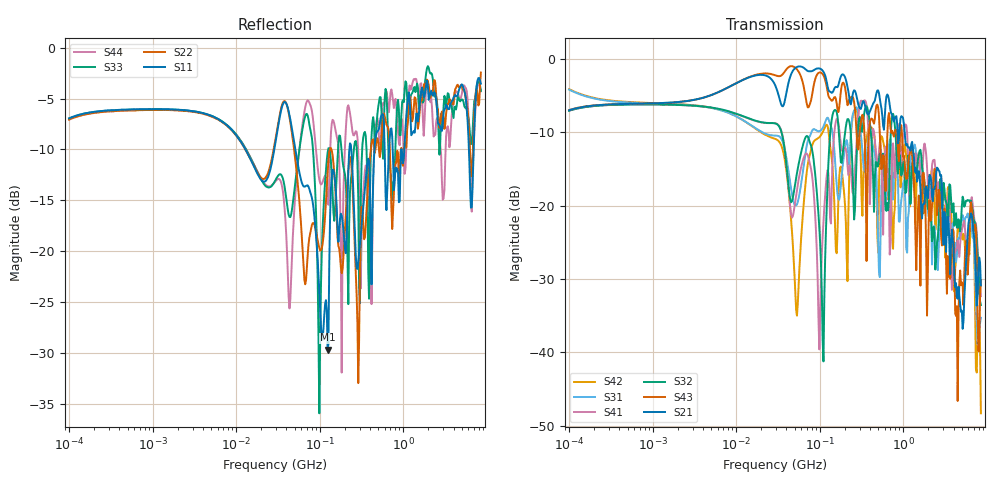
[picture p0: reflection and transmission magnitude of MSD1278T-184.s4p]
# MHz S MA R 50
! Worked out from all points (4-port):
!   498 points, 100 kHz to 8.5 GHz, reference 50 ohm
!   strongest paths, dB at 100 kHz, 1.698 MHz, 29.49 MHz, 500.7 MHz, 8.5 GHz:
!     S21: -7.0, -6.0, -3.7, -4.3, -30.9
!     S43: -7.0, -6.0, -2.3, -6.7, -30.2
!     S32: -7.1, -6.3, -8.8, -14.6, -33.5
!     S41: -7.1, -6.3, -8.8, -14.0, -32.3
!     S31: -4.2, -6.2, -10.5, -24.9, -35.3
!     S42: -4.2, -6.2, -10.9, -26.3, -48.3
!   lowest |S11| = -29.7 dB at 124.3 MHz (marker M1), VSWR 1.07, Z = 53.3 - j0.646 ohm
!   |S11| at or under -10 dB: 51.1 MHz to 226.3 MHz (175.2 MHz wide, 126 % of centre); 238.3 MHz to 452.9 MHz (214.6 MHz wide, 62.1 % of centre); 6.109 GHz to 6.966 GHz (857.5 MHz wide, 13.1 % of centre)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
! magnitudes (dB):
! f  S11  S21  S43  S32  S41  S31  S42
! 100 kHz  -6.9  -7.0  -7.0  -7.1  -7.1  -4.2  -4.2
! 31.58 MHz  -7.9  -4.7  -2.4  -9.0  -9.0  -10.5  -11.1
! 53.4 MHz  -10.9  -1.1  -1.5  -15.6  -17.8  -19.9  -35.0
! 124.3 MHz  -29.7  -3.8  -4.6  -16.9  -15.2  -8.0  -9.2
! 4.383 GHz  -4.8  -32.5  -33.7  -23.0  -25.8  -26.8  -25.3
! 6.612 GHz  -15.7  -21.3  -20.3  -20.1  -18.9  -23.0  -21.4
! 8.5 GHz  -3.5  -30.9  -30.2  -33.5  -32.3  -35.3  -48.3
